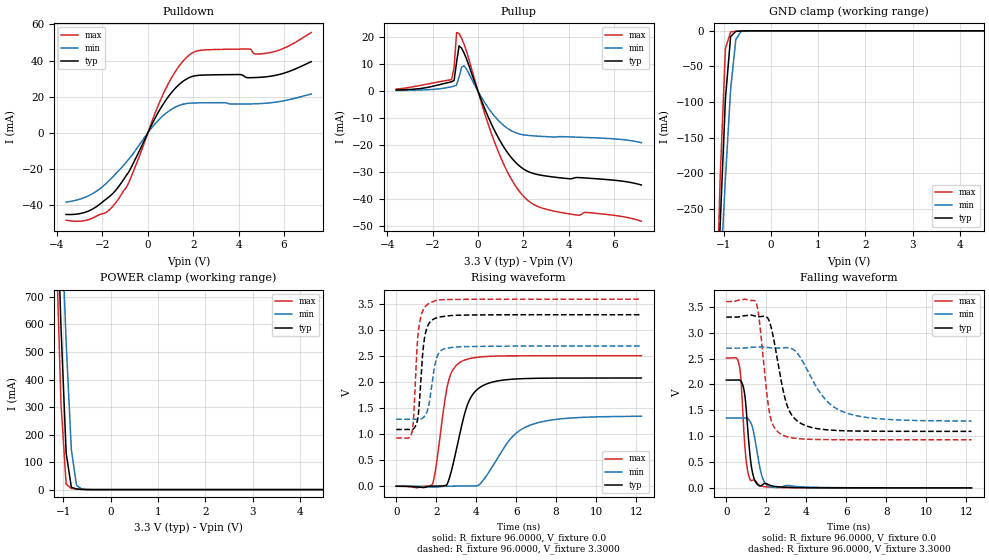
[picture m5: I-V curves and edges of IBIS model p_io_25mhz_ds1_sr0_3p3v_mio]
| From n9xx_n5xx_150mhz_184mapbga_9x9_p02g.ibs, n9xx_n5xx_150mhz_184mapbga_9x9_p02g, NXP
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[Model] p_io_25mhz_ds1_sr0_3p3v_mio
|   Model p_io_25mhz_ds1_sr0_3p3v_mio
| This model was characterised for following simulation conditions:
| External (pad) voltage:
|   - Typ: 3.3V,   - Min: 2.7V,   - Max: 3.6V
| Library cells for typ/min/max conditions are connected as defined below:
|  pad - External Pad
|  ipp_do_lv - Core Input
|  ipp_obe_lv - Output Buffer Enable
|  IOGC - NC
|  REFH3V3 - REFH3V3
|  REFL3V3 - REFL3V3
|  ZI - NC
|  abut_ncal_vddio[1] - vddio
|  abut_ncal_vddio[2] - vddio
|  abut_ncal_vddio[3] - vssio
|  abut_ncal_vddio[4] - vddio
|  abut_ncal_vddio[5] - vddio
|  abut_ncal_vddio[6] - vssio
|  abut_pcal_vddio[1] - vssio
|  abut_pcal_vddio[2] - vssio
|  abut_pcal_vddio[3] - vddio
|  abut_pcal_vddio[4] - vssio
|  abut_pcal_vddio[5] - vssio
|  abut_pcal_vddio[6] - vddio
|  ipp_do_1p8v - ipp_do_1p8v
|  ipp_dse_lv - vdd_lv
|  ipp_eftd_lv - NC
|  ipp_ina_mux_vddio - NC
|  ipp_ina_mux_vddio[0] - NC
|  ipp_ina_mux_vddio[1] - NC
|  ipp_ina_r0_vddio - NC
|  ipp_ina_r0a_vddio - NC
|  ipp_ina_r0b_vddio - NC
|  ipp_ina_r0c_vddio - NC
|  ipp_ina_r0d_vddio - NC
|  ipp_ina_r0e_vddio - NC
|  ipp_ina_r0f_vddio - NC
|  ipp_ina_r300_vddio - NC
|  ipp_ina_r300a_vddio - NC
|  ipp_ina_r300b_vddio - NC
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Model_type I/O
Polarity   Non-Inverting
Enable   Active-High
Vinl =   0.9900V
Vinh =   2.3100V
Vmeas =  1.6500V
Cref =   30.0000pF
Rref =   1.0000M
Vref =   3.3000V
C_comp   1.2813pF   1.2310pF   1.3501pF
|C_comp_pullup   0.5365pF   0.5679pF   0.5152pF
|C_comp_pulldown   0.6537pF   0.6898pF   0.6250pF
[Model Spec]
| variable   typ   min   max
Vinh   2.3100V   1.8900V   2.5200V
Vinl   0.9900V   0.8100V   1.0800V
[Temperature Range]   25.0000   0.1250k   -40.0000
[Voltage Range]   3.3000V   2.7000V   3.6000V
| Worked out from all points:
|   slope of the pulldown table from 0 to 0.495 V, typ, clamps not added: 40.9 ohm
|   slope of the pullup table from 0 to 0.495 V, typ, clamps not added: 47.8 ohm
|   GND clamp passes 1 mA (typ) near -0.74 V on its own axis
|   POWER clamp passes 1 mA (typ) near -0.62 V on its own axis
|   rising waveform, R_fixture 96.0000, V_fixture 0.0: 20-80 % time 832ps typ, 1.56ns min, 566ps max; typ from 0 V to 2.08 V
|   rising waveform, R_fixture 96.0000, V_fixture 3.3000: 20-80 % time 277ps typ, 354ps min, 247ps max; typ from 1.09 V to 3.3 V
|   falling waveform, R_fixture 96.0000, V_fixture 0.0: 20-80 % time 291ps typ, 387ps min, 253ps max; typ from 2.08 V to 0 V
|   falling waveform, R_fixture 96.0000, V_fixture 3.3000: 20-80 % time 721ps typ, 1.49ns min, 452ps max; typ from 3.3 V to 1.09 V
[Pulldown]
|Voltage   I(typ)   I(min)   I(max)
-3.6V     -44.98mA   -38.16mA   -48.14mA
-2.5V     -42.45mA   -33.96mA   -47.35mA
-1.84V    -36.56mA   -27.93mA   -43.93mA
-1.4V     -31.43mA   -22.35mA   -38.33mA
-850mV    -21.79mA   -14.63mA   -27.72mA
800mV     18.2mA     10.89mA    24.65mA
1.35V     26.4mA     15.02mA    36.44mA
1.9V      30.96mA    16.49mA    43.72mA
4.43V     30.51mA    16mA       46.38mA
4.76V     30.6mA     16.11mA    43.52mA
5.31V     31.15mA    16.54mA    44.2mA
7.2V      39.37mA    21.51mA    55.42mA
[Pullup]
|Voltage   I(typ)   I(min)   I(max)
-3.6V     375.6uA    207.2uA    723.4uA
-1.16V    3.421mA    1.609mA    4.222mA
-1.05V    3.932mA    1.826mA    8.69mA
-940mV    10.66mA    2.21mA     21.59mA
-830mV    16.71mA    5.23mA     21.25mA
-720mV    15.83mA    8.864mA    19.49mA
-610mV    14.01mA    9.303mA    17.31mA
820mV     -16.02mA   -10.13mA   -20.77mA
1.48V     -24.67mA   -14.68mA   -32.64mA
2.03V     -28.89mA   -16.19mA   -39.05mA
3.35V     -31.77mA   -16.98mA   -44.33mA
7.2V      -34.69mA   -19.05mA   -48.09mA
[GND_clamp]
|Voltage   I(typ)   I(min)   I(max)
-3.6V     -5.285A    -4.099A    -6.854A
-1.18V    -466mA     -495.3mA   -458.9mA
-1.07V    -271.1mA   -348.5mA   -204.6mA
-960mV    -95.66mA   -207.9mA   -24.82mA
-850mV    -8.126mA   -81.84mA   -1.536mA
-740mV    -740.4uA   -12.14mA   -755uA
-630mV    -283.6uA   -928.1uA   -319.7uA
-300mV    -497.8nA   -2.865uA   -109.5nA
7.2V      0A         0A         0A
[POWER_clamp]
|Voltage   I(typ)   I(min)   I(max)
-3.6V     14.48A     12.95A     16.35A
-1.16V    1.177A     1.535A     951.2mA
-1.05V    598.3mA    1.032A     318mA
-940mV    134.2mA    537.3mA    19.98mA
-830mV    8.694mA    145.4mA    4.231mA
-720mV    2.123mA    15.37mA    2.22mA
-610mV    848.6uA    1.85mA     839.5uA
7.2V      0A         0A         0A
[Ramp]
| variable   typ   min   max
dV/dt_r  1.2496/0.8324n   0.8075/1.5600n   1.5065/0.5659n
dV/dt_f  1.3247/0.7214n   0.8453/1.4881n   1.6022/0.4514n
R_load = 96.0000
[Rising Waveform]
R_fixture= 96.0000
V_fixture= 0.0
V_fixture_min= 0.0
V_fixture_max= 0.0
|time   V(typ)   V(min)   V(max)
0s        3.132nV    106.7nV    10.54nV
1.807ns   2.816mV    -15.11mV   35.49mV
1.999ns   3.481mV    -16.46mV   391.3mV
2.59ns    76.86mV    1.8mV      1.984V
3.271ns   1.157V     1.82mV     2.401V
3.788ns   1.744V     2.705mV    2.466V
4.8ns     2.003V     368.4mV    2.502V
5.786ns   2.059V     940.9mV    2.509V
6.862ns   2.076V     1.197V     2.51V
12.27ns   2.083V     1.346V     2.511V
[Rising Waveform]
R_fixture= 96.0000
V_fixture= 3.3000
V_fixture_min= 2.7000
V_fixture_max= 3.6000
|time   V(typ)   V(min)   V(max)
0s        1.092V     1.289V     929.6mV
789.3ps   1.091V     1.289V     1.04V
877.5ps   1.11V      1.289V     1.365V
1.025ns   1.212V     1.289V     2.568V
1.162ns   1.627V     1.289V     3.126V
1.368ns   2.714V     1.326V     3.407V
1.639ns   3.132V     1.576V     3.515V
2.013ns   3.239V     2.449V     3.577V
2.434ns   3.27V      2.647V     3.591V
12.27ns   3.3V       2.7V       3.6V
[Falling Waveform]
R_fixture= 96.0000
V_fixture= 0.0
V_fixture_min= 0.0
V_fixture_max= 0.0
|time   V(typ)   V(min)   V(max)
0s        2.083V     1.349V     2.511V
611.8ps   2.085V     1.348V     2.427V
720.3ps   2.068V     1.348V     2.155V
825.3ps   1.984V     1.349V     1.453V
959.6ps   1.673V     1.351V     652.8mV
1.103ns   977.2mV    1.327V     262.1mV
1.319ns   277.3mV    1.153V     149.4mV
1.675ns   37.81mV    396.2mV    43.86mV
2.397ns   28.8mV     9.769mV    10.22mV
12.27ns   275.8nV    18.43uV    15.51nV
[Falling Waveform]
R_fixture= 96.0000
V_fixture= 3.3000
V_fixture_min= 2.7000
V_fixture_max= 3.6000
|time   V(typ)   V(min)   V(max)
0s        3.3V       2.7V       3.6V
1.49ns    3.316V     2.721V     3.584V
1.642ns   3.307V     2.725V     3.266V
2.171ns   3.2V       2.709V     1.426V
2.773ns   2.014V     2.707V     1.029V
3.118ns   1.516V     2.705V     979.6mV
3.579ns   1.285V     2.589V     951.9mV
4.878ns   1.128V     1.746V     933.1mV
5.894ns   1.104V     1.463V     930.7mV
12.27ns   1.092V     1.291V     929.6mV
